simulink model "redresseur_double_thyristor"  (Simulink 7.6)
settings: Solver=ode23tb  StartTime=0.0  StopTime=0.04  RelTol=1e-4
InitFcn:
  | clear all
  | clc
  | delete *.mat
StopFcn:
  | close all
  | load Ug_Us.mat
  | subplot 211
  | plot(x(1,:),x(3,:))
  | grid
  | title('commande gâchette')
  | xlabel('temps')
  | axis([0 0.04 -0.2 1.2])
  | 
  | 
  | subplot 212
  | plot(x(1,:),x(2,:))
  | grid
  | title('Tension aux bornes de la charge')
  | axis([0 0.04 -20 120])
  | xlabel('temps')
  | 
  | 
  | delete *.mat
libraries: powerlib x7, powerlib_extras x1

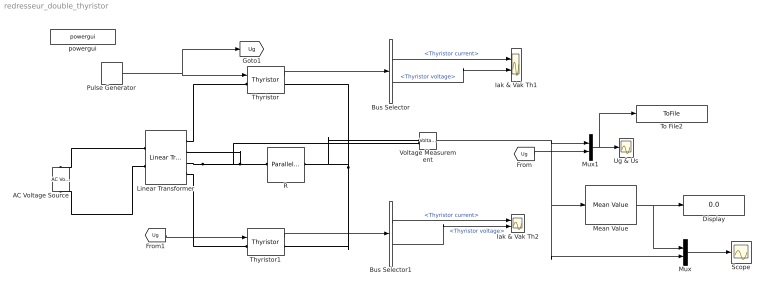
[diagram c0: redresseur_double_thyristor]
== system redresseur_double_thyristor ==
  AC Voltage Source : powerlib/Electrical Sources/AC Voltage Source  DialogController=POWERSYS.PowerSysDialog  SystemSampleTime=-1  Amplitude=100  Phase=0  Frequency=60  SampleTime=0  Measurements=None
  Bus Selector : BusSelector  OutputSignals=Thyristor current,Thyristor voltage
  Bus Selector1 : BusSelector  OutputSignals=Thyristor current,Thyristor voltage
  Display : Display
  Iak & Vak Th1 : Scope  NumInputPorts=2
  Iak & Vak Th2 : Scope  NumInputPorts=2
  Linear Transformer : powerlib/Elements/Linear Transformer  DialogController=POWERSYS.PowerSysDialog  PhysicalDomain=powersysdomain  SubClassName=unknown  LeftPortType=p1  RightPortType=p1  LConnTagsString=a|b  RConnTagsString=A|B|C|D  UNITS=pu  NominalPower=[ 250e6 60 ]  winding1="[100/sqrt(2)  0.002  0.08 ]"  winding2="[100/sqrt(2)  0.002  0.08 ]"  ThreeWindings=on  winding3="[100/sqrt(2)  0.002 0.08 ]"  RmLm=[ 500 500 ]  Measurements=None  DataType=off
  Mean Value : powerlib_extras/Measurements/Mean Value  DialogController=POWERSYS.PowerSysDialog  SystemSampleTime=-1  Period=1/60
  Mux : Mux  Inputs=2
  Mux1 : Mux  Inputs=2
  Pulse Generator : DiscretePulseGenerator  PulseType=Time based  Period=1/120  PulseWidth=2  PhaseDelay=0.2/120
  R : powerlib/Elements/Parallel RLC Branch  DialogController=POWERSYS.PowerSysDialog  PhysicalDomain=powersysdomain  SubClassName=unknown  LeftPortType=p1  RightPortType=p1  LConnTagsString=a  RConnTagsString=__new0  BranchType=R  Resistance=1  Inductance=1e-3  SetiL0=off  InitialCurrent=0  Capacitance=1e-6  Setx0=off  InitialVoltage=0  Measurements=None
  Scope : Scope
  Thyristor : powerlib/Power Electronics/Thyristor  DialogController=POWERSYS.PowerSysDialog  SystemSampleTime=-1  Ron=0.001  Lon=0  Vf=0.8  IC=0  Rs=500  Cs=250e-9  Measurements=on
  Thyristor1 : powerlib/Power Electronics/Thyristor  DialogController=POWERSYS.PowerSysDialog  SystemSampleTime=-1  Ron=0.001  Lon=0  Vf=0.8  IC=0  Rs=500  Cs=250e-9  Measurements=on
  To File2 : ToFile  Filename=Ug_Us  MatrixName=x
  Ug & Us : Scope
  Voltage Measurement : powerlib/Measurements/Voltage Measurement  DialogController=POWERSYS.PowerSysDialog  SystemSampleTime=-1  PhasorSimulation=off  OutputType=Complex  PSBequivalent=0
  powergui : powerlib/powergui  Priority=2  SystemSampleTime=-1  SimulationMode=Continuous  SampleTime=0  frequency=60  SPID=off  DisableSnubberDevices=off  DisableRonSwitches=off  DisableVfSwitches=off  SwTol=0  Interpol=off  frequencyindice=0  echomessages=off  HookPort=off  DisplayEquations=off  FunctionMessages=off  EnableUseOfTLC=off  x0status=blocks  RestoreLinks=warning  ResistiveCurrentMeasurement=off  Frange=logspace(0,3,50)  Ylog=off  Xlog=off  ShowGrid=off  save=off  variable=ZData  ZoomFFT=on  StartTime=0.0  cycles=1  DisplayStyle=off  fundamental=60  FreqAxis=off  MaxFrequency=1000  frequencyindicesteady=1  RmsSteady=1  display=off  Ts=0  methode=off
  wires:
  Bus Selector/1 -> Iak & Vak Th1/1  "<Thyristor current>"
  Bus Selector/2 -> Iak & Vak Th1/2  "<Thyristor voltage>"
  Thyristor/1 -> Bus Selector/1
  Pulse Generator/1 -> Thyristor/1, [Ug]
  Voltage Measurement/1 -> Mean Value/1, Mux/2, Mux1/1
  Mean Value/1 -> Display/1, Mux/1
  Mux/1 -> Scope/1
  [Ug] -> Thyristor1/1
  Thyristor1/1 -> Bus Selector1/1
  Bus Selector1/1 -> Iak & Vak Th2/1  "<Thyristor current>"
  Bus Selector1/2 -> Iak & Vak Th2/2  "<Thyristor voltage>"
  [Ug] -> Mux1/2
  Mux1/1 -> Ug & Us/1, To File2/1
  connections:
  R/LConn1 -- Thyristor/RConn1 -- Thyristor1/RConn1 -- Voltage Measurement/LConn1
  Linear Transformer/LConn1 -- AC Voltage Source/RConn1
  Linear Transformer/LConn2 -- AC Voltage Source/LConn1
  Linear Transformer/RConn2 -- Linear Transformer/RConn3 -- R/RConn1 -- Voltage Measurement/LConn2
  Linear Transformer/RConn1 -- Thyristor/LConn1
  Linear Transformer/RConn4 -- Thyristor1/LConn1
